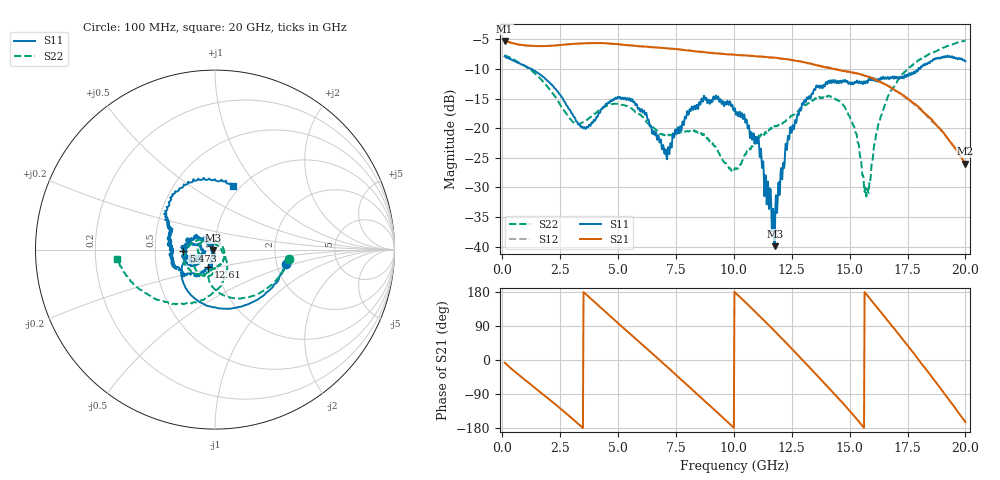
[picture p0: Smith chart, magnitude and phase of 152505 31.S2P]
!  2-Port S-parameters saved by WinCal
! VAR MeasName=S-Parameters (CALIBRATED_DATA) read from VNA (N5230C)
! VAR MeasDate=4/10/2015 9:31:25 AM
! VAR NAME=152505 31
! VAR FILENAME=152505 31.S2P
! VAR DATE=4/10/2015 9:31:25 AM
! VAR PHYS_PORTS=1,2
# Hz S DB R 50
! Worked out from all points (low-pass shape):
!   801 points, 100 MHz to 20 GHz, reference 50 ohm
!   highest |S21| = -5.28 dB at 100 MHz (marker M1); lowest = -26.0 dB at 20 GHz (marker M2)
!   |S21| within 3 dB of the highest: start of sweep to 12.06 GHz
!   lowest |S11| = -39.9 dB at 11.77 GHz (marker M3), VSWR 1.02, Z = 49 - j0.239 ohm
!   |S11| at or under -10 dB: 1.265 GHz to 17.97 GHz (16.71 GHz wide, 174 % of centre); 18.02973 GHz to 18.0419 GHz (12.17 MHz wide, 0.0675 % of centre)
!   |S22| runs from -31.6 to -5.2 dB; largest |S21 - S12| = 0.0068
!   S11 on the Smith chart (normalised r, x): 100 MHz: 2.26, -0.42; 5.473 GHz: 0.70, -0.01; 12.61 GHz: 0.91, -0.18; 20 GHz: 0.93, +0.76
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1e8  -7.85 -11.1  -5.28 -7.1  -5.30 -7.0  -7.66 -7.4
8.71125e8  -9.30 -72.0  -5.97 -47.2  -5.98 -47.1  -9.26 -45.4
1.7915e9  -11.40 -127.8  -6.16 -92.1  -6.14 -92.1  -12.26 -84.1
3.43325e9  -19.70 -157.9  -5.70 -176.8  -5.70 -176.8  -19.11 -94.1
4.552625e9  -15.79 -147.4  -5.69 121.7  -5.71 121.6  -16.13 -108.4
5.473e9  -15.10 -178.2  -6.01 71.5  -5.97 71.4  -16.42 -139.2
6.741625e9  -21.19 167.2  -6.41 2.7  -6.40 2.5  -20.69 -162.9
7.11475e9  -25.25 -170.3  -6.52 -18.1  -6.52 -17.9  -21.20 -163.0
8.383375e9  -16.23 -160.3  -7.06 -88.1  -7.02 -88.0  -20.53 171.5
1.005e10  -16.70 157.0  -7.62 178.3  -7.63 177.9  -26.74 26.6
1.106988e10  -21.54 138.3  -7.89 118.4  -7.86 118.3  -21.24 -63.1
1.176638e10  -39.92 -166.0  -8.10 76.3  -8.11 76.1  -19.59 -89.4
1.23385e10  -21.31 -105.1  -8.37 40.2  -8.43 39.7  -18.38 -100.9
1.261212e10  -19.71 -112.2  -8.56 22.6  -8.55 22.8  -17.69 -105.5
1.338325e10  -14.17 -134.1  -9.20 -26.9  -9.16 -26.8  -15.29 -126.2
1.480112e10  -11.84 -173.4  -10.39 -119.9  -10.34 -121.0  -16.50 171.3
1.529862e10  -12.07 178.7  -10.77 -155.1  -10.67 -155.5  -20.96 140.8
1.57215e10  -12.03 175.7  -11.24 173.8  -11.18 173.7  -31.55 58.1
1.669162e10  -11.67 164.2  -12.92 100.5  -13.03 99.3  -14.34 -77.5
1.783588e10  -10.71 151.4  -15.96 12.6  -16.21 11.6  -8.97 -122.1
1.875625e10  -8.28 127.1  -19.50 -60.9  -19.55 -60.5  -6.97 -145.8
2e10  -8.71 73.9  -25.98 -164.2  -26.05 -163.0  -5.20 -174.7
